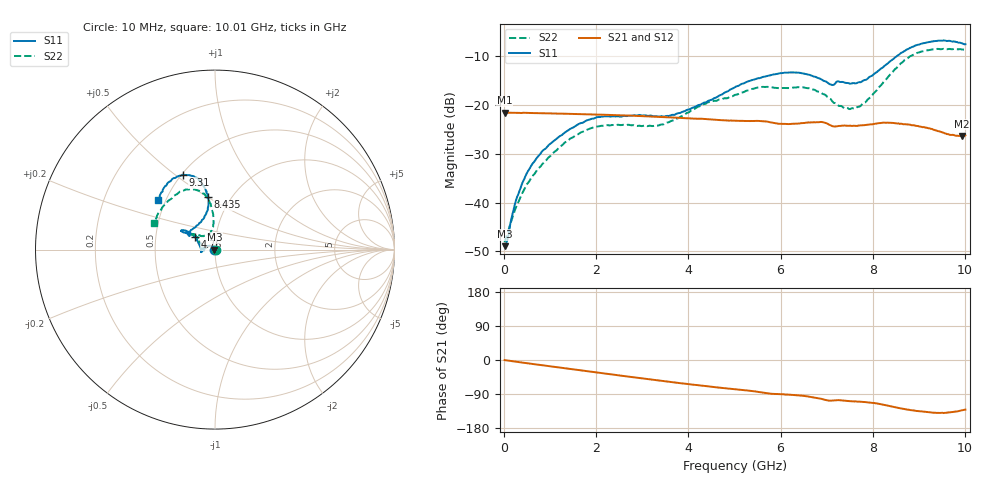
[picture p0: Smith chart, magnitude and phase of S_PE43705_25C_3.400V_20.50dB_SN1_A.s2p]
! Device ID: PE43705
! Serial: 1
! Insertion: A
! Impedance: 50 ohm
! Temp: 25C
! VDD: 3.400V
! Attenuation Step: 20.50dB
#  Hz  S  RI  R  50
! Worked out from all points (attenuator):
!   401 points, 10 MHz to 10.01 GHz, reference 50 ohm
!   highest |S21| = -21.53 dB at 10 MHz (marker M1); lowest = -26.3 dB at 9.935 GHz (marker M2)
!   lowest |S11| = -48.9 dB at 10 MHz (marker M3), VSWR 1.01, Z = 49.6 + j0.0395 ohm
!   |S11| at or under -10 dB: start of sweep to 8.517 GHz
!   |S22| runs from -48.1 to -8.5 dB; largest |S21 - S12| = 0.00085
!   S11 on the Smith chart (normalised r, x): 10 MHz: 0.99, +0.00; 4.76 GHz: 0.79, +0.11; 8.435 GHz: 0.79, +0.50; 9.31 GHz: 0.51, +0.53; 10.01 GHz: 0.45, +0.31
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1e7  -0.00356 0.000397  0.0838 -0.000339  0.0839 -0.000329  0.00393 0.000388
6e7  -0.00336 0.00219  0.0836 -0.00164  0.0836 -0.00163  0.00421 0.00192
2.85e8  -0.00556 0.0101  0.083 -0.00711  0.083 -0.00704  0.00212 0.00935
5.6e8  -0.0132 0.0184  0.0818 -0.0138  0.0818 -0.0137  -0.00462 0.0164
1.01e9  -0.0344 0.0214  0.0786 -0.0241  0.0787 -0.024  -0.0238 0.0187
1.685e9  -0.0652 0.00822  0.0715 -0.0377  0.0715 -0.0376  -0.0523 0.00856
2.16e9  -0.0763 -0.00673  0.065 -0.0461  0.0649 -0.0461  -0.0614 -0.00152
3.36e9  -0.0759 -0.00645  0.0442 -0.0615  0.0444 -0.0614  -0.0615 0.00839
4.76e9  -0.111 0.0705  0.0191 -0.0673  0.0193 -0.0673  -0.0969 0.0654
5.01e9  -0.1268 0.0854  0.0153 -0.0675  0.0154 -0.0676  -0.1044 0.0731
5.535e9  -0.1583 0.1027  0.00648 -0.0685  0.00655 -0.0683  -0.122 0.0897
5.985e9  -0.1821 0.1087  -0.000235 -0.0644  3.8e-05 -0.0642  -0.1195 0.0893
6.685e9  -0.1747 0.0952  -0.0094 -0.0658  -0.00958 -0.0659  -0.1199 0.0809
7.11e9  -0.1403 0.0801  -0.018 -0.0586  -0.0182 -0.0587  -0.0808 0.0768
7.585e9  -0.1018 0.1341  -0.0202 -0.058  -0.0201 -0.0579  -0.0361 0.0849
7.885e9  -0.0609 0.1761  -0.0233 -0.0585  -0.0233 -0.0586  -0.0164 0.1125
8.36e9  -0.0351 0.275  -0.0344 -0.0565  -0.0345 -0.0563  -0.0115 0.2018
8.435e9  -0.038 0.2925  -0.0361 -0.0549  -0.0362 -0.055  -0.0147 0.2198
8.86e9  -0.089 0.3859  -0.0423 -0.0457  -0.0422 -0.0461  -0.0729 0.3166
9.31e9  -0.1765 0.4158  -0.0425 -0.0368  -0.0422 -0.0369  -0.1702 0.3316
9.935e9  -0.3075 0.301  -0.0328 -0.0354  -0.0331 -0.0353  -0.3252 0.1801
1.001e10  -0.3162 0.2777  -0.0321 -0.0371  -0.0325 -0.037  -0.341 0.1504
